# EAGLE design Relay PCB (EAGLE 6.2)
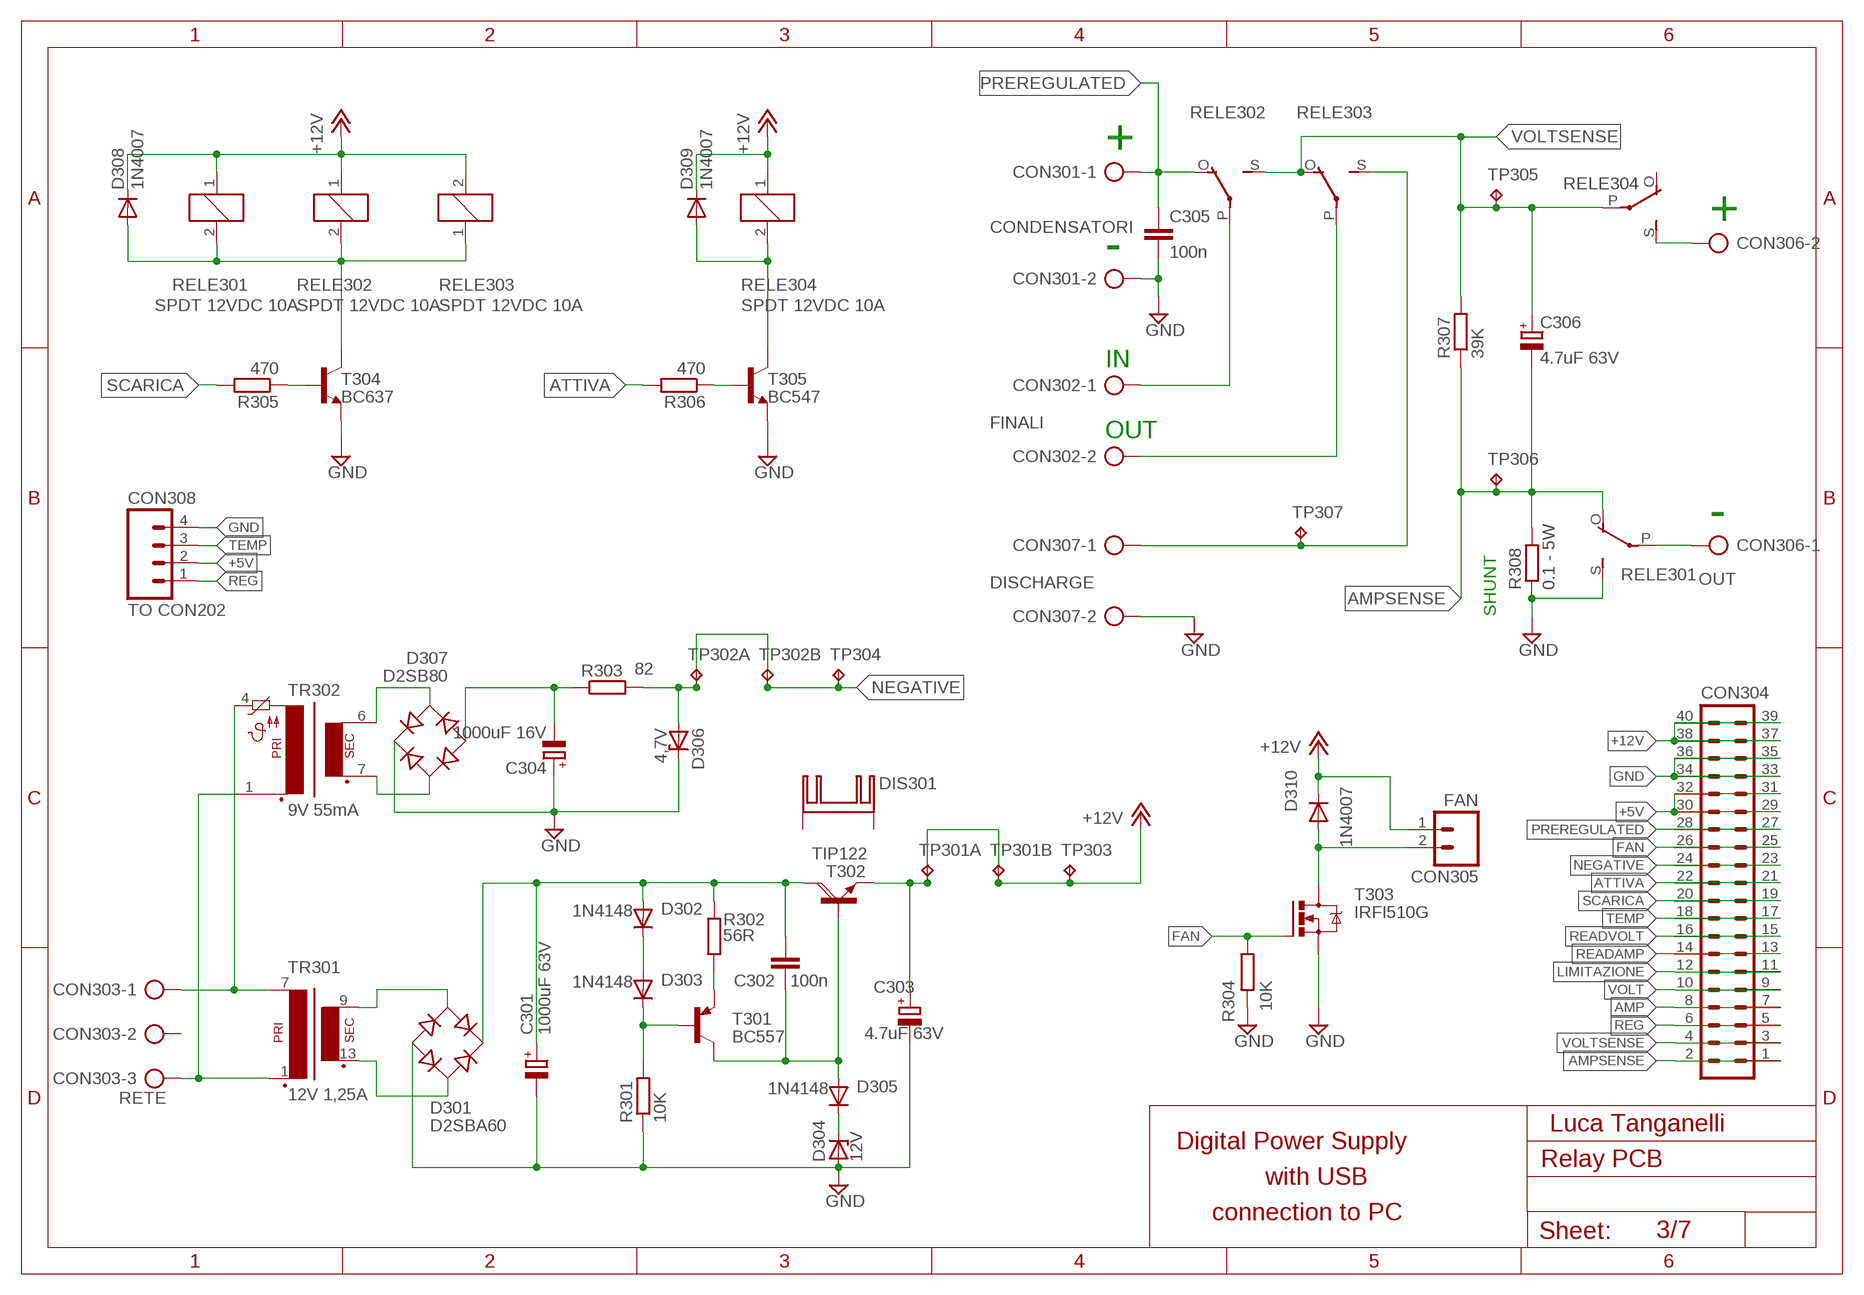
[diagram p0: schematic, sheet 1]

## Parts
C301  1000uF 63V  CPOL-EUE5-10.5  [E5-10,5]
C302  100n  C-EU050-024X044  [C050-024X044]
C303  4.7uF 63V  CPOL-EUE2.5-5  [E2,5-5]
C304  1000uF 16V  CPOL-EUE5-10.5  [E5-10,5]
C305  100n  C-EU050-024X044  [C050-024X044]
C306  4.7uF 63V  CPOL-EUE2.5-5  [E2,5-5]
CON301  CONDENSATORI  AK500/2  [AK500/2]
CON302  FINALI  AK500/2  [AK500/2]
CON303  RETE  AK500/3  [AK500/3]
CON304  ML40  [ML40]
CON305  FAN  M02  [02P]
CON306  OUT  AK500/2  [AK500/2]
CON307  DISCHARGE  AK500/2  [AK500/2]
CON308  TO CON202  M04  [04P]
D301  D2SBA60  RECTIFIER-GBU4S  [GBU4S]
D302  1N4148  1N4148DO35-7  [DO35-7]
D303  1N4148  1N4148DO35-7  [DO35-7]
D304  12V  BZX85  [DO41Z10]
D305  1N4148  1N4148DO35-7  [DO35-7]
D306  4,7V  1N4728  [DO41Z10]
D307  D2SB80  RECTIFIER-RB1A  [RB1A]
D308  1N4007  1N4004  [DO41-10]
D309  1N4007  1N4004  [DO41-10]
D310  1N4007  1N4004  [DO41-10]
DIS301  MIO  [MIO]
R301  10K  R-EU_0207/10  [0207/10]
R302  56R  R-EU_0207/10  [0207/10]
R303  82  R-EU_0207/10  [0207/10]
R304  10K  R-EU_0207/10  [0207/10]
R305  470  R-EU_0207/10  [0207/10]
R306  470  R-EU_0207/10  [0207/10]
R307  39K  R-EU_0309/V  [0309V]
R308  0.1 - 5W  R-EU_0921/26  [0921/26]
RELE301  SPDT 12VDC 10A  ZF112  [ZF112]
RELE302  SPDT 12VDC 10A  ZF112  [ZF112]
RELE303  SPDT 12VDC 10A  ZF112  [ZF112]
RELE304  SPDT 12VDC 10A  ZF112  [ZF112]
T301  BC557  [TO92-EBC]
T302  TIP122  [TO220AV]
T303  IRFI510G  IRF520  [TO220BV]
T304  BC637  -NPN-TO92-ECB  [TO92-ECB]
T305  BC547  BC547-NPN-TO92-CBE  [TO92-CBE]
TP301  TP2  [TP2]
TP302  TP2  [TP2]
TP303  TP  [TP1]
TP304  TP  [TP1]
TP305  TP  [TP1]
TP306  TP  [TP1]
TP307  TP  [TP1]
TR301  12V 1,25A  PE5420D09477  [PE54]
TR302  9V 55mA  VN20.10  [VN2010]

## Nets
+5V: CON304.29 CON304.30 CON304.31 CON304.32 CON308.2
+12V: CON304.37 CON304.38 CON304.39 CON304.40 CON305.1 D308.C D309.C D310.C RELE301.1 RELE302.1 RELE303.2 RELE304.1 TP301.P$2 TP303.P$1(TP)
AC_0: D301.AC2 TR301.13(S3)
AC_18: D301.AC1 TR301.9(S4)
AMP: CON304.7 CON304.8
AMPSENSE: C306.- CON304.1 CON304.2 R307.1 R308.P$2 RELE301.O(2:O) TP306.P$1(TP)
ATTIVA: CON304.21 CON304.22 R306.2
DISCHARGE: CON307.1 RELE303.S(2:S) TP307.P$1(TP)
FAN: CON304.25 CON304.26 R304.1 T303.G
GND: C301.- C303.- C304.+ C305.2 CON301.2 CON304.33 CON304.34 CON304.35 CON304.36 CON307.2 CON308.4 D301.- D304.A D306.C D307.+ R301.1 R304.2 R308.P$1 RELE301.S(2:S) T303.S T304.E T305.E
LIMITAZIONE: CON304.11 CON304.12
N$1: CON302.1 RELE302.P(2:P)
N$2: CON303.1 TR301.7(P1) TR302.4
N$3: CON303.3 TR301.1(P2) TR302.1
N$8: CON306.1 RELE301.P(2:P)
N$9: D306.A R303.2 TP302.P$1
N$10: C303.+ T302.E TP301.P$1
N$15: D304.C D305.C
N$24: D307.AC2 TR302.6
N$26: D307.AC1 TR302.7
N$27: CON306.2 RELE304.S(2:S)
N$28: C304.- D307.- R303.1
N$43: C302.1 D305.A T301.C T302.B
N$44: C301.+ C302.2 D301.+ D302.A R302.1 T302.C
N$46: D302.C D303.A
N$47: D303.C R301.2 T301.B
N$49: R302.2 T301.E
N$55: R305.1 T304.B
N$57: D308.A RELE301.2 RELE302.2 RELE303.1 T304.C
N$62: R306.1 T305.B
N$64: D309.A RELE304.2 T305.C
N$94: CON305.2 D310.A T303.D
NEGATIVE: CON304.23 CON304.24 TP302.P$2 TP304.P$1(TP)
POWER_OUT: CON302.2 RELE303.P(2:P)
PREREGULATED: C305.1 CON301.1 CON304.27 CON304.28 RELE302.O(2:O)
READAMP: CON304.13 CON304.14
READVOLT: CON304.15 CON304.16
REG: CON304.5 CON304.6 CON308.1
SCARICA: CON304.19 CON304.20 R305.2
TEMP: CON304.17 CON304.18 CON308.3
VOLT: CON304.9 CON304.10
VOLTSENSE: C306.+ CON304.3 CON304.4 R307.2 RELE302.S(2:S) RELE303.O(2:O) RELE304.P(2:P) TP305.P$1(TP)
Unconnected: CON303.2 DIS301.P$1(K) DIS301.P$2(K) RELE304.O(2:O)

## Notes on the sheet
- +
- +
- -
- IN
- OUT
- -
- SHUNT
- Luca Tanganelli
- Digital Power Supply
- with USB
- connection to PC
- 3/7

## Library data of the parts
C301 C303 C304 C306 = #-rcl:CPOL-EU: POLARIZED CAPACITOR, European symbol
C302 C305 = #-rcl:C-EU: CAPACITOR, European symbol
CON301 CON302 CON306 CON307 = #-con-ptr500:AK500/2: CONNECTOR; OC_FARNELL: unknown; OC_NEWARK: unknown
CON303 = #-con-ptr500:AK500/3: CONNECTOR; OC_FARNELL: unknown; OC_NEWARK: unknown
CON304 = #-con-ml:ML40: HARTING; OC_FARNELL: unknown; OC_NEWARK: unknown
CON305 = #-con-amp-quick:M02: AMP QUICK CONNECTOR; OC_FARNELL: unknown; OC_NEWARK: unknown
CON308 = #-con-amp-quick:M04: AMP QUICK CONNECTOR; OC_FARNELL: unknown; OC_NEWARK: unknown
D301 D307 = #-rectifier:RECTIFIER-: Rectifier
D302 D303 D305 = #-diode:1N4148: DIODE
D304 = #-diode:BZX85: Z DIODE
D306 = #-diode:1N4728: Z DIODE
D308-D310 = #-diode:1N4004: DIODE
DIS301 = #-heatsink:MIO
R301-R308 = #-rcl:R-EU_: RESISTOR, European symbol
RELE301-RELE304 = relay:ZF112: RELAY 1 x switch; OC_FARNELL: unknown; OC_NEWARK: unknown
T301 = #-transistor-pnp:BC557*: PNP Transistror
T302 = #-transistor-power:TIP122
T303 = #-transistor-power:IRF520: HEXFET Power MOSFET
T304 T305 = #-transistor:*-NPN-: NPN Transistror BF959 corrected 2008.03.06
TP301 TP302 = #-testpad:TP2: Test pad
TP303-TP307 = #-testpad:TP: Test pad
TR301 = #-trafo:PE5420D09477
TR302 = #-trafo:VN20.10

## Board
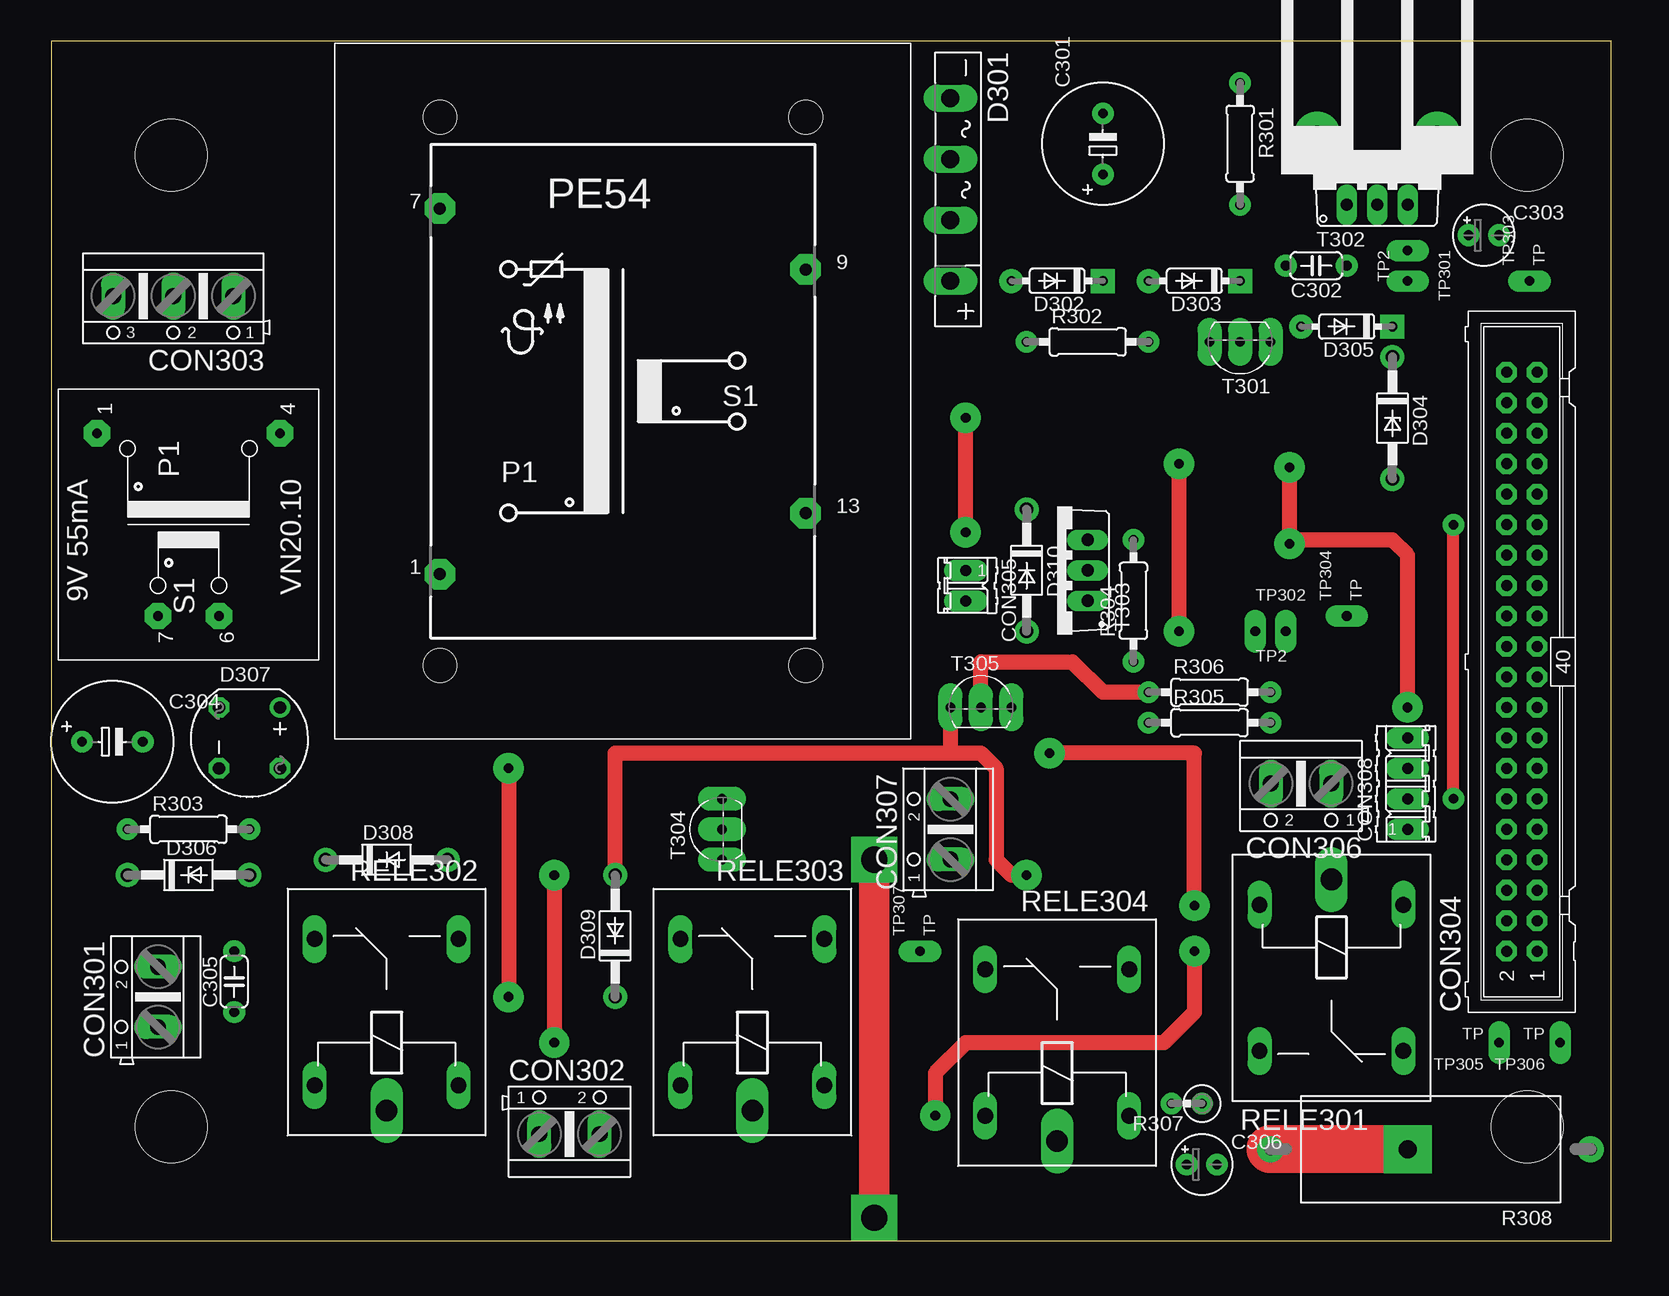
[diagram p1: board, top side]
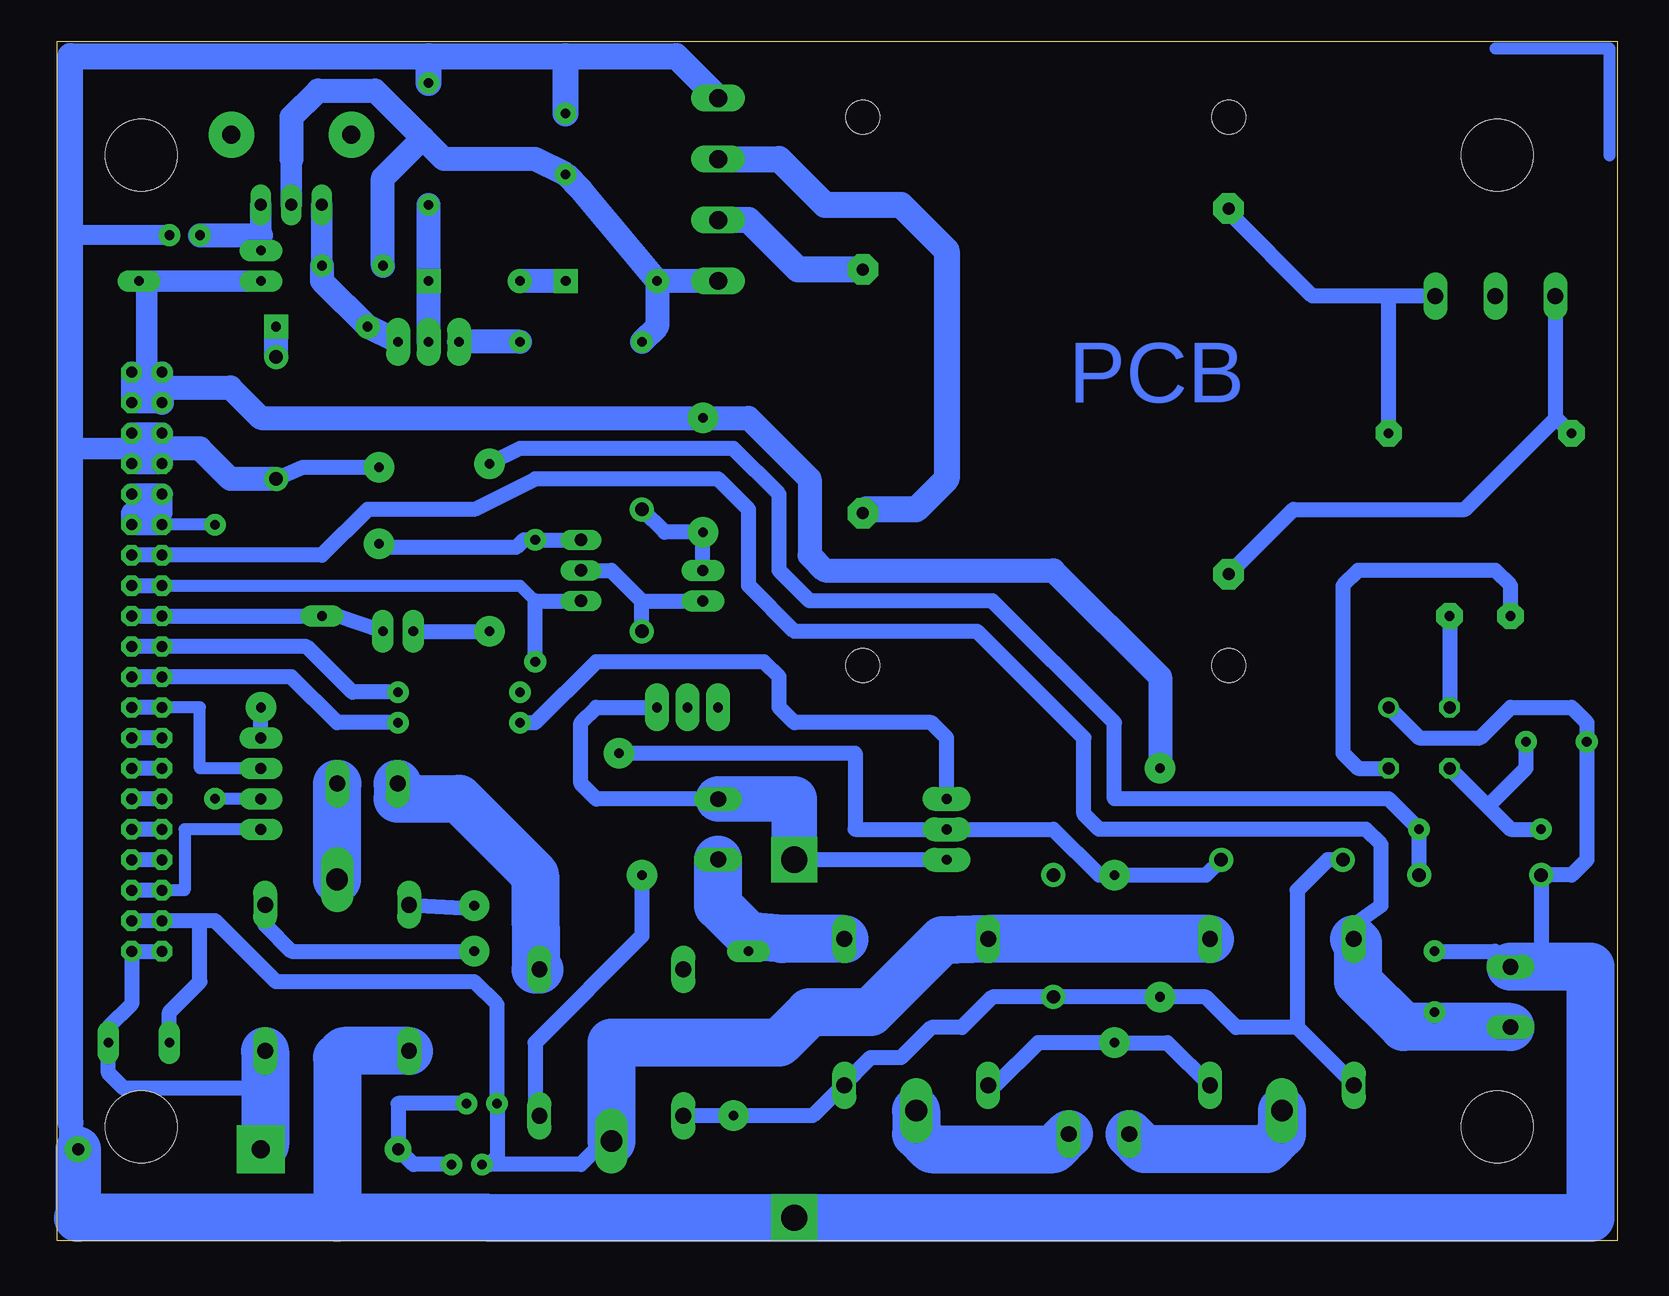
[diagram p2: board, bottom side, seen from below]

Size 130 x 100 mm. Coordinates in mm from the lower left corner, seen from the top.
Outline: 130,100 0,100 0,0 130,0 130,100
Copper layers (1*16): Top 0.035mm / dielectric 1.5mm / Bottom 0.035mm
Design rules: minimum track width 10mil, minimum drill 24mil, track to track 8mil, track to pad 8mil, pad to pad 8mil, via to via 8mil, smd to smd 8mil, copper to edge 40mil, drill to drill 8mil, minimum pad ring 10mil, minimum via ring 8mil, stop-mask expansion 4mil, vias tented up to drill 0mil, thermal gap 10mil
Holes 6 mm at 123,9.5 123,90.5 10,90.5 10,9.5

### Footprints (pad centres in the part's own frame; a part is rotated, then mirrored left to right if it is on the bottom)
E5-10,5 = drill 0.8 pad 1.8: + -2.54,0; - 2.54,0
C050-024X044 = drill 0.8 pad 1.8: 1 -2.54,0; 2 2.54,0
E2,5-5 = drill 0.8 pad 1.8: + -1.27,0; - 1.27,0
AK500/2 = drill 1.321 pad 1.7 long: 1 -2.515,0; 2 2.515,0
AK500/3 = drill 1.321 pad 1.7 long: 1 -5.004,0; 2 0,0; 3 5.004,0
ML40 = drill 0.914 pad 1.7 octagon: 1 -24.13,-1.27; 2 -24.13,1.27; 3 -21.59,-1.27; 4 -21.59,1.27; 5 -19.05,-1.27; 6 -19.05,1.27; 7 -16.51,-1.27; 8 -16.51,1.27; 9 -13.97,-1.27; 10 -13.97,1.27; 11 -11.43,-1.27; 12 -11.43,1.27; 13 -8.89,-1.27; 14 -8.89,1.27; 15 -6.35,-1.27; 16 -6.35,1.27; 17 -3.81,-1.27; 18 -3.81,1.27; 19 -1.27,-1.27; 20 -1.27,1.27; 21 1.27,-1.27; 22 1.27,1.27; 23 3.81,-1.27; 24 3.81,1.27; 25 6.35,-1.27; 26 6.35,1.27; 27 8.89,-1.27; 28 8.89,1.27; 29 11.43,-1.27; 30 11.43,1.27; 31 13.97,-1.27; 32 13.97,1.27; 33 16.51,-1.27; 34 16.51,1.27; 35 19.05,-1.27; 36 19.05,1.27; 37 21.59,-1.27; 38 21.59,1.27; 39 24.13,-1.27; 40 24.13,1.27
02P = drill 0.914 pad 1.8 long: 1 -1.27,0; 2 1.27,0
04P = drill 0.914 pad 1.8 long: 1 -3.81,0; 2 -1.27,0; 3 1.27,0; 4 3.81,0
GBU4S = drill 1.499 pad 1.7 long: + 7.62,0; - -7.62,0; AC1 2.54,0; AC2 -2.54,0
DO35-7 = drill 0.813 pad 2: A 3.81,0 | drill 0.813 pad 2 square: C -3.81,0
DO41Z10 = drill 1.118 pad 2: A 5.08,0; C -5.08,0
RB1A = drill 1.016 pad 1.7: + -2.54,2.54 | drill 1.016 pad 1.7 octagon: - 2.54,-2.54; AC1 2.54,2.54; AC2 -2.54,-2.54
DO41-10 = drill 1.118 pad 2: A 5.08,0; C -5.08,0
MIO = drill 1.5 pad 3.81: P$1 3.3,-5; P$2 3.3,5
0207/10 = drill 0.8 pad 1.8: 1 -5.08,0; 2 5.08,0
0309V = drill 0.8 pad 1.8: 1 -1.27,0; 2 1.27,0
0921/26 = drill 1 pad 2.184: P$1 -13.335,0; P$2 13.335,0
ZF112 = drill 1.321 long: 1 -6.096,5.994; 2 -6.096,-5.994; O 6.096,5.994; S 6.096,-5.994 | drill 1.803 long: P -8.204,0
TO92-EBC = drill 0.813 pad 2 long: B 0,-1.27; C -2.54,-1.27; E 2.54,-1.27
TO220AV = drill 1.016 pad 1.7 long: B -2.54,-2.54; C 0,-2.54; E 2.54,-2.54
TO220BV = drill 1.016 pad 1.7 long: D 0,-2.54; G -2.54,-2.54; S 2.54,-2.54
TO92-ECB = drill 0.813 pad 2 long: B 2.54,0; C 0,0; E -2.54,0
TO92-CBE = drill 0.813 pad 2 long: B 0,0; C -2.54,0; E 2.54,0
TP2 = drill 0.8 pad 1.778 long: P$1 -1.27,0; P$2 1.27,0
TP1 = drill 0.8 pad 1.778 long: P$1 0,0
PE54 = drill 1 pad 2.54 octagon: 1 -15.24,-15.24; 7 -15.24,15.24; 9 15.24,10.16; 13 15.24,-10.16 | hole 2.8: -15.24,-22.86; -15.24,22.86; 15.24,22.86; 15.24,-22.86
VN2010 = drill 0.8 pad 2.184 octagon: 1 -7.62,-7.62; 4 -7.62,7.62; 6 7.62,2.54; 7 7.62,-2.54

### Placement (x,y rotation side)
C301  87.63,91.44 90 top
C302  105.41,81.28 180 top
C303  119.38,83.82 0 top
C304  5.08,41.59 0 top
C305  15.24,21.59 90 top
C306  95.89,6.35 0 top
CON301  8.89,20.32 90 top
CON302  43.18,8.89 0 top
CON303  10.16,78.74 180 top
CON304  122.54,48.26 90 top
CON305  76.2,54.61 270 top
CON306  104.14,38.1 180 top
CON307  74.93,34.29 90 top
CON308  113.03,38.1 90 top
D301  74.93,87.63 270 top
D302  83.82,80.01 180 top
D303  95.25,80.01 180 top
D304  111.76,68.58 270 top
D305  107.95,76.2 180 top
D306  11.43,30.48 0 top
D307  16.51,41.91 270 top
D308  27.94,31.75 0 top
D309  46.99,25.4 90 top
D310  81.28,55.88 270 top
DIS301  110.49,88.9 90 top
R301  99.06,91.44 270 top
R302  86.36,74.93 0 top
R303  11.43,34.29 0 top
R304  90.17,53.34 90 top
R305  96.52,43.18 0 top
R306  96.52,45.72 0 top
R307  94.61,11.43 180 top
R308  114.94,7.62 180 top
RELE301  106.68,21.91 270 top
RELE302  27.94,19.05 90 top
RELE303  58.42,19.05 90 top
RELE304  83.82,16.51 90 top
T301  99.06,73.66 180 top
T302  110.49,88.9 0 top
T303  83.82,55.88 90 top
T304  55.88,34.29 90 top
T305  77.47,44.45 0 top
TP301  113.03,81.28 270 top
TP302  101.6,50.8 0 top
TP303  123.19,80.01 90 top
TP304  107.95,52.07 90 top
TP305  120.65,16.51 180 top
TP306  125.73,16.51 180 top
TP307  72.39,24.13 90 top
TR301  47.62,70.8 0 top
TR302  11.43,59.69 270 top

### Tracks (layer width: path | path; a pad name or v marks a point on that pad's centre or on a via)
+5V  (via drill 0.8 pad 1.78)
  Top 1.016: v116.84,36.83 v116.84,59.69
  Bottom 1.016: CON308.2 v116.84,36.83 | v116.84,59.69 CON304.30
  Bottom 1.778: CON304.30 CON304.29 123.81,60.64 121.28,60.64 121.28,62.23 CON304.32 CON304.31
+12V  (via drill 0.8 pad 2.54)
  Top 1.27: v38.1,39.37 v38.1,20.32 | v76.2,59.05 v76.2,68.58 | v95.25,24.13 95.25,19.05 92.71,16.51 76.2,16.51 73.66,13.97 v73.66,10.41
  Bottom 1.27: RELE302.1 21.95,13.06 26.67,17.78 | 64.77,12.7 62.23,15.24 59.69,15.24 57.15,17.78 54.61,17.78 52.07,20.32 D309.C v38.1,20.32 34.29,20.32 31.75,17.78 26.67,17.78 | 64.77,12.7 64.67,12.7 RELE303.2 | D308.C 24.13,31.75 26.67,29.21 26.67,17.78 | 64.77,12.7 67.06,10.41 v73.66,10.41 RELE304.1 | CON305.1 v76.2,59.05 79.38,59.05 D310.C | RELE301.1 112.67,26.31 110.49,24.13 v95.25,24.13
  Bottom 1.778: TP301.P$2 122.56,80.01 | 122.56,80.01 TP303.P$1 | CON304.38 CON304.37 CON304.39 122.56,71.14 | CON304.38 CON304.40 | 122.56,71.14 122.56,71.12 | 122.56,71.14 122.56,80.01 | CON304.38 121.92,70.5 121.92,71.12
  Bottom 2: CON304.38 121.27,70.47 121.92,71.12 115.57,71.12 113.03,68.58 v76.2,68.58 72.39,68.58 67.31,63.5 67.31,57.15 66.04,55.88 46.99,55.88 38.1,46.99 v38.1,39.37
AC_0
  Bottom 2.184: D301.AC2 69.85,90.17 66.04,86.36 59.69,86.36 55.88,82.55 55.88,63.5 58.42,60.96 62.55,60.96 TR301.13
AC_18
  Bottom 2.184: TR301.9 68.26,80.96 72.39,85.09 D301.AC1
AMP
  Bottom 1.27: CON304.8 CON304.7
AMPSENSE  (via drill 1.5 pad 4)
  Top 4: v113.03,7.62 R308.P$2
  Bottom 1.27: CON304.2 CON304.1 123.81,19.7 125.73,17.78 TP306.P$1 125.73,13.97 124.46,12.7 112.67,12.7 | R307.1 101.6,11.43 R308.P$2 100.33,6.35 C306.-
  Bottom 4: RELE301.O 112.67,12.7 112.67,7.98 v113.03,7.62
ATTIVA
  Bottom 1.27: CON304.21 CON304.22 109.22,49.53 105.41,45.72 R306.2
DISCHARGE
  Bottom 1.27: TP307.P$1 72.39,25.4
  Bottom 4: RELE303.S 69.6,25.15 72.39,25.4 74.93,27.94 CON307.1
FAN
  Bottom 1.016: CON304.26 91.44,54.61 90.17,53.34
  Bottom 1.27: CON304.25 CON304.26 | T303.G 90.17,53.34 R304.1
GND  (via drill 0.8 pad 2.54, 2.2 pad 3.81)
  Top 1.27: v103.19,64.45 v103.19,58.1 103.5,58.42 111.76,58.42 113.03,57.15 v113.03,44.45
  Top 2.54: v68.58,31.75 v68.58,1.91
  Bottom 1.27: C305.2 10.19,24.13 CON301.2 | D307.+ 16.51,41.91 11.43,41.91 8.89,44.45 3.81,44.45 2.54,43.18 C304.+ 2.54,31.75 3.81,30.48 D306.C 6.35,22.84 | T303.S R304.2 91.12,58.42 91.76,57.78 102.87,57.78 v103.19,58.1 | v103.19,64.45 109.54,64.45 D304.A | T304.E v68.58,31.75 | CON307.2 85.06,36.8 86.36,38.1 86.36,43.18 85.09,44.45 T305.E | CON308.4 v113.03,44.45
  Bottom 1.676: C303.- 128.91,83.82
  Bottom 1.778: CON304.36 CON304.34 CON304.33 | CON304.35 CON304.36 | CON304.36 122.23,66.35 122.54,66.04 128.91,66.04
  Bottom 1.93: 128.91,9.84 128.91,8.26 R308.P$1
  Bottom 2: D304.A 115.57,63.5 118.11,66.04 121.92,66.04 122.23,66.35
  Bottom 2.184: 128.91,9.84 128.91,66.04 128.91,83.82 128.91,98.74 99.06,98.74 | 99.06,98.74 87.63,98.74 | 87.63,98.74 78.42,98.74 D301.- | C301.- 87.63,98.74 | R301.1 99.06,98.74
  Bottom 3.81: CON307.2 68.58,36.8 v68.58,31.75 | 106.68,1.91 113.03,1.91 | 128.27,1.91 R308.P$1
  Bottom 4: CON301.2 6.35,22.84 2.25,22.84 2.22,22.86 2.22,1.91 v68.58,1.91 93.98,1.91 106.68,1.91 | 106.68,1.91 128.27,1.91 | RELE301.S 106.11,15.81 106.68,15.24 106.68,1.91
LIMITAZIONE
  Bottom 1.27: CON304.12 CON304.11
N$1
  Bottom 4: RELE302.P 27.94,8.89 29.21,7.62 39.4,7.62 CON302.1
N$2
  Bottom 1.27: CON303.1 19.05,78.74 | 19.05,78.74 25.4,78.74 32.38,85.72 TR301.7 | TR302.4 19.05,78.74
N$3
  Bottom 1.27: CON303.3 5.16,68.66 5.08,68.58 | 5.08,68.58 TR302.1 | TR301.1 26.99,60.96 12.7,60.96 5.08,68.58
N$4  (via drill 0.8 pad 3.81)
  other vias: 10,90.5
N$5  (via drill 0.8 pad 3.81)
  other vias: 123,90.5
N$6  (via drill 0.8 pad 3.81)
  other vias: 10,9.5
N$7  (via drill 0.8 pad 3.81)
  other vias: 123,9.5
N$8
  Bottom 4: RELE301.P 106.68,38.08 CON306.1
N$9  (via drill 0.8 pad 2.54)
  Top 1.27: v93.98,50.8 v93.98,64.77
  Bottom 1.27: D306.A R303.2 19.05,36.83 41.91,36.83 41.91,43.18 52.07,53.34 67.31,53.34 69.85,55.88 69.85,62.23 73.66,66.04 91.44,66.04 v93.98,64.77 | TP302.P$1 v93.98,50.8
N$10
  Bottom 1.778: T302.E 113.03,83.82 TP301.P$1
  Bottom 2: C303.+ 113.03,83.82
N$11  (via drill 0.8 pad 2.54)
  other vias: 32.38,93.66
N$12  (via drill 0.8 pad 2.54)
  other vias: 62.87,93.66
N$13  (via drill 0.8 pad 2.54)
  other vias: 62.87,47.94
N$14  (via drill 0.8 pad 2.54)
  other vias: 32.38,47.94
N$15
  Bottom 2: D304.C D305.C
N$16
  Bottom 1.016: 0.64,90.49 0.64,99.38 10.16,99.38
N$24
  Bottom 1.27: TR302.6 D307.AC2
N$26
  Bottom 1.27: TR302.7 8.89,54.61 10.16,55.88 21.59,55.88 22.86,54.61 22.86,40.64 21.59,39.37 D307.AC1
N$27
  Bottom 4: RELE304.S 90.13,22.58 90.17,29.92 90.17,30.48 96.52,36.83 101.62,36.85 CON306.2
N$28
  Bottom 1.27: D307.- 10.79,36.2 | 10.79,36.2 8.89,34.29 R303.1 | C304.- 7.62,39.37 10.79,36.2
N$43
  Bottom 1.778: C302.1 T302.B
  Bottom 2: T301.C D305.A 107.95,80.01 C302.1
N$44
  Bottom 1.778: T302.C 110.49,90.17
  Bottom 2: D301.+ D302.A | D302.A 80.01,76.2 R302.1 | D302.A 86.36,87.63 C301.+ 90.17,90.17 97.79,90.17 99.54,91.92 | 99.54,91.92 103.5,95.89 108.27,95.89 110.49,93.66 110.49,90.17 | C302.2 102.87,88.58 99.54,91.92
N$46
  Bottom 2: D302.C D303.A
N$47
  Bottom 2: T301.B D303.C R301.2
N$49
  Bottom 2: R302.2 T301.E
N$55
  Bottom 1.27: T304.B 55.88,41.91 57.15,43.18 68.58,43.18 69.85,44.45 69.85,46.99 71.12,48.26 85.09,48.26 90.17,43.18 R305.1
N$57  (via drill 0.8 pad 2.54)
  Top 1.27: v41.91,30.48 v41.91,16.51 | v95.25,27.94 95.25,40.64 v83.19,40.64
  Bottom 1.27: RELE303.1 51.82,12.95 48.26,16.51 v41.91,16.51 37.49,16.51 RELE302.2 | D308.A 34.29,30.48 v41.91,30.48 43.18,30.48 46.99,34.29 T304.C 63.5,34.29 63.5,40.64 v83.19,40.64 | RELE301.2 95.5,27.69 v95.25,27.94
N$62
  Top 1.27: T305.B 77.47,48.26 85.09,48.26 87.63,45.72 R306.1
N$64  (via drill 0.8 pad 2.54)
  Top 1.27: D309.A 46.99,40.64 74.93,40.64 | T305.C 74.93,40.64 | 74.93,40.64 77.47,40.64 78.74,39.37 78.74,31.75 80.01,30.48 v81.28,30.48
  Bottom 1.27: v81.28,30.48 81.28,25.4 90.17,16.51 90.17,10.77 RELE304.2
N$94
  Bottom 1.27: T303.D 83.82,55.88 81.28,53.34 | 81.28,53.34 CON305.2 | D310.A 81.28,53.34
NEGATIVE
  Bottom 1.27: CON304.23 CON304.24 TP304.P$1 106.68,52.07 TP302.P$2
POWER_OUT
  Bottom 4: RELE303.P 58.42,8.89 57.15,7.62 46.97,7.62 CON302.2
PREREGULATED
  Bottom 1.27: 17.8,17.8 16.48,17.8 C305.1 | RELE302.O 21.95,26.31 19.68,27.94 19.68,33.02 20.95,34.29 43.18,34.29 44.45,35.56 44.45,41.91 53.34,50.8 68.58,50.8 72.39,54.61 72.39,60.96 74.93,63.5 90.17,63.5 95.25,60.96 104.14,60.96 107.95,57.15 CON304.28 CON304.27
  Bottom 4: CON301.1 17.8,17.8 21.59,21.59 21.59,24.79 RELE302.O
READAMP
  Bottom 1.27: CON304.14 CON304.13
READVOLT
  Bottom 1.27: CON304.16 CON304.15
REG
  Bottom 1.016: CON308.1 119.38,34.29 119.38,29.21 CON304.6
  Bottom 1.27: CON304.6 CON304.5
SCARICA
  Bottom 1.27: CON304.19 CON304.20 110.49,46.99 106.68,43.18 R305.2
TEMP
  Bottom 1.016: CON308.3 118.11,39.37 118.11,44.45 CON304.18
  Bottom 1.27: CON304.18 CON304.17
VOLT
  Bottom 1.27: CON304.10 CON304.9
VOLTSENSE
  Bottom 1.27: CON304.3 CON304.4 118.11,26.67 | RELE303.O 53.34,26.06 | RELE304.P 84.4,8.31 86.36,6.35 93.98,6.35 | 93.98,6.35 C306.+ | 93.98,6.35 93.34,6.99 R307.2 93.34,19.68 95.25,21.59 111.76,21.59 116.84,26.67 118.11,26.67 | TP305.P$1 120.65,19.05 118.11,21.59 118.11,26.67
  Bottom 4: RELE304.P 83.82,16.51 69.85,16.51 67.31,19.05 62.23,19.05 56.24,25.04 RELE303.O RELE302.S

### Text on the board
Bottom: PCB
